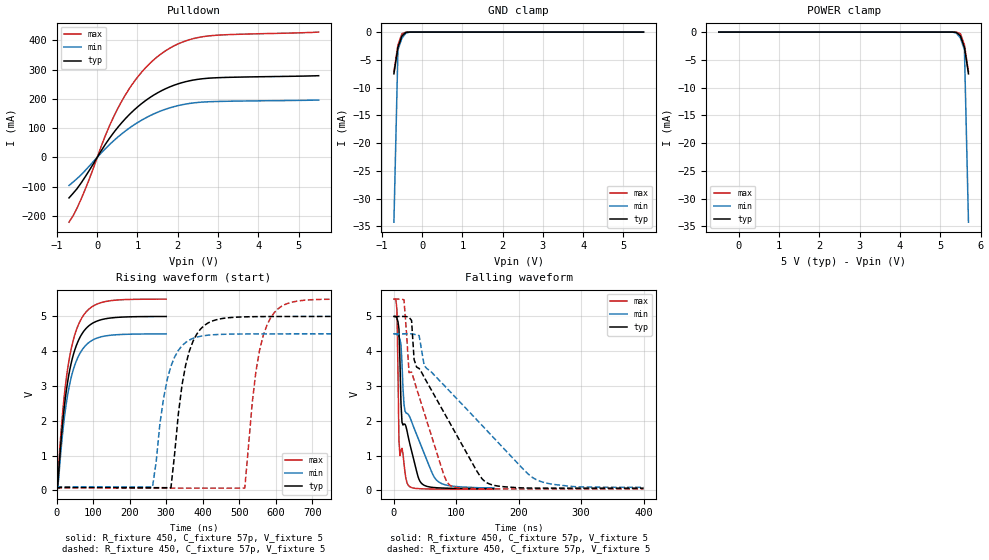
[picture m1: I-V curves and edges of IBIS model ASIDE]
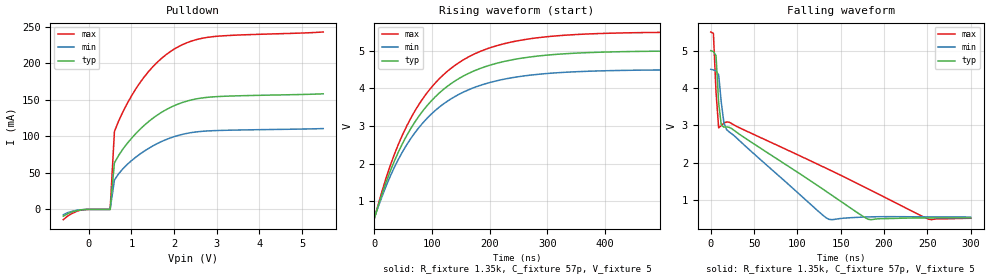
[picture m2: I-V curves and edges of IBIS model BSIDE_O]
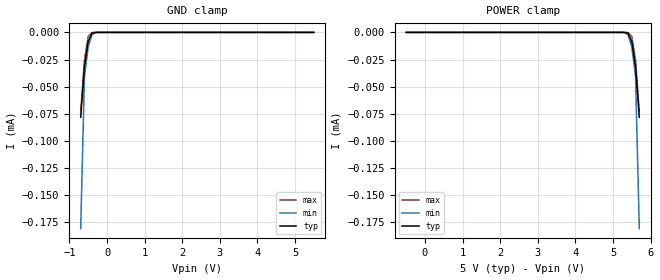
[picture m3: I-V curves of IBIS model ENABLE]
[IBIS Ver]   3.2
[Comment Char]   |_char
| VDD nom: 5v, min: 4.5v, max:5.5v
[File name]   pca9507_a_5.ibs
[File Rev]   1
[Date]   Sep 19, 2008 3:12:36 PM
[Source]
Generated using IBISToolkit at NXP Tempe by Seshadri Venkataramanan
[Notes]
[Disclaimer]
(C) Copyright 2007 NXP Semiconductors
All rights reserved
NXP Semiconductors (NXP) does not warrant that this model and any other
accompanying information (Model) accurately or fully represents the
operating characteristics and specifications of the semiconductor
products to which the Model relates.  Moreover, the Model is furnished
on an "as is" and with "all faults" basis, and without support or
warranty of any kind.  NXP disclaims all warranties, whether expressed
or implied or statutory, including without limitation all implied
warranties of non-infringement, merchantability and fitness for any
purpose, and those arising from a course of dealing or usage of trade.
NXP does not convey any license under its or any third party's patents,
copyrights or other intellectual property or proprietary rights.
You and your company assume any and all risks and liability arising out
of the application or use of the Model.
In no event shall NXP be liable for any direct, indirect, special,
consequential or incidental damages, however caused, whether in
warranty, contract or tort (including negligence), strict liability or
other legal theory, including, without limitation, for lost profits,
business interruption, or corruption or loss of data or information,
arising out of or in connection with the use of or the inability to use
the Model, even if NXP has been advised of the possibility of such
damages.
NXP provides the Model as a courtesy to our customers. You and your
company shall not distribute, convey, sell, or give the Model to anyone
else without receiving prior written permission from NXP.
NXP reserves the right to make changes without notice to the Model to
improve reliability, function, or design.
Please be aware that your receipt and subsequent use of the Model shall
serve as acceptance of these terms and conditions.  If you do not
accept these terms, return or destroy the Model immediately.
[Copyright]
2008
| SO8
[Component]   PCA9507D
Si_location Pin
Timing_location Pin
[Manufacturer]   NXP
[Package]
R_pkg   4.81E-02   4.14E-02   5.47E-02
L_pkg   1.88n   1.54n   2.21n
C_pkg   4.49E-13   4.17E-13   4.81E-13
[Pin] signal_name   model_name   R_pin   L_pin   C_pin
1   VCCA   POWER   5.47E-02  2.21E-09  4.81E-13
2   SCLA   ASIDE   4.14E-02  1.54E-09  4.20E-13
3   SDAA   ASIDE   4.14E-02  1.55E-09  4.20E-13
4   GND   GND   5.47E-02  2.21E-09  4.80E-13
5   EN   ENABLE   5.47E-02  2.21E-09  4.78E-13
6   SDAB   BSIDE_I/O   4.14E-02  1.55E-09  4.17E-13
7   SCLB   BSIDE_I/O   4.14E-02  1.54E-09  4.17E-13
8   VCCB   POWER   5.47E-02  2.21E-09  4.79E-13
| TSSOP8
[Component]   PCA9507AD
Si_location Pin
Timing_location Pin
[Manufacturer]   NXP
[Package]
R_pkg   33.7m   30.1m   37.3m
L_pkg   1.74n   1.67n   1.81n
C_pkg   0.428p   0.422p   0.434p
[Pin] signal_name   model_name   R_pin   L_pin   C_pin
1   VCCA   POWER   37.3m   1.81nH   0.428pF
2   SCLA   ASIDE   30.1m   1.67nH   0.422pF
3   SDAA   ASIDE   30.1m   1.67nH   0.428pF
4   GND   GND   37.3m   1.81nH   0.434pF
5   EN   ENABLE   37.3m   1.81nH   0.428pF
6   SDAB   BSIDE_I/O   30.1m   1.67nH   0.422pF
7   SCLB   BSIDE_I/O   30.1m   1.67nH   0.428pF
8   VCCB   POWER   37.3m   1.81nH   0.434pF
[Model Selector]   BSIDE_I/O
BSIDE_I   Bside as Input
BSIDE_O   Bside as Output
| Models and submodels in the file (4): ASIDE (I/O_open_drain), BSIDE_O (Open_drain), ENABLE (Input), BSIDE_I (Input)
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[Model]   ASIDE
Model_type I/O_open_drain
Vinh=3.5
Vinl=1.5
Vref=5
Vmeas=2.5
Rref=450
Cref=57p
C_comp   5.2p   5p   5.4p
[Temperature Range] 27   85   -40
[Voltage Range]   5   4.5   5.5
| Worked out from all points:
|   slope of the pulldown table from 0 to 0.75 V, typ, clamps not added: 5.37 ohm
|   GND clamp passes 1 mA (typ) near -0.52 V on its own axis
|   falling waveform, R_fixture 450, C_fixture 57p, V_fixture 5: 20-80 % time 20.5ns typ, 37.9ns min, 3.61ns max; typ from 5 V to 0.049 V
|   falling waveform, R_fixture 450, C_fixture 57p, V_fixture 5: 20-80 % time 85.9ns typ, 140ns min, 47.2ns max; typ from 5 V to 0.061 V
|   rising waveform, R_fixture 450, C_fixture 57p, V_fixture 5: 20-80 % time 39.7ns typ, 39.8ns min, 39.6ns max; typ from 0.048 V to 5 V
|   rising waveform, R_fixture 450, C_fixture 57p, V_fixture 5: 20-80 % time 40.5ns typ, 40.9ns min, 40.5ns max; typ from 0.061 V to 5 V
[Pulldown]
-700mV    -138.9mA   -96.33mA   -222.1mA
-600mV    -123.5mA   -84.89mA   -200.6mA
-400mV    -87.94mA   -59.92mA   -143mA
-200mV    -45.56mA   -30.51mA   -75.7mA
200mV     44.01mA    29.24mA    73.36mA
600mV     117mA      79.31mA    190.1mA
800mV     146.6mA    100.3mA    235.7mA
1.1V      183.6mA    126.9mA    291mA
1.6V      228.3mA    159.8mA    355.5mA
2.1V      255.4mA    179.8mA    393.6mA
2.7V      270.2mA    189.8mA    414.5mA
5.5V      279.4mA    196.1mA    428.8mA
[GND Clamp]
-700mV    -7.514mA   -34.24mA   -7.128mA
-600mV    -2.754mA   -3.204mA   -2.306mA
-500mV    -688.4uA   -1.069mA   -295.4uA
-400mV    -56.78uA   -166.7uA   -8.032uA
-200mV    -26.65nA   -203.8nA   -760.1pA
5.5V      375pA      669.7pA    343.7pA
[POWER Clamp]
-500mV    375pA      669.7pA    343.7pA
5.2V      -26.65nA   -203.8nA   -760.1pA
5.4V      -56.78uA   -166.7uA   -8.032uA
5.5V      -688.4uA   -1.069mA   -295.4uA
5.6V      -2.754mA   -3.204mA   -2.306mA
5.7V      -7.514mA   -34.24mA   -7.128mA
[Falling Waveform]
R_fixture=450
C_fixture=57p
V_fixture=5
V_fixture_min=4.5
V_fixture_max=5.5
0s        5V         4.5V       5.5V
4.848ns   4.951V     4.489V     5.198V
8.081ns   4.643V     4.412V     1.43V
9.697ns   3.689V     4.343V     994mV
12.93ns   1.961V     3.654V     1.206V
16.16ns   1.905V     2.473V     768mV
22.63ns   1.566V     2.192V     153.7mV
42.02ns   250.3mV    1.352V     45.07mV
69.49ns   72.05mV    272.6mV    34.02mV
160ns     48.56mV    67.26mV    32.13mV
[Falling Waveform]
R_fixture=450
C_fixture=57p
V_fixture=5
V_fixture_min=4.5
V_fixture_max=5.5
0s        5V         4.5V       5.5V
16.16ns   5V         4.5V       5.477V
24.24ns   4.976V     4.5V       3.385V
28.28ns   4.886V     4.499V     3.401V
36.36ns   3.543V     4.471V     2.919V
48.48ns   3.251V     3.591V     2.235V
88.89ns   1.96V      2.859V     155.3mV
153.5ns   178.3mV    1.631V     39.97mV
234.3ns   62.63mV    258.8mV    39.21mV
400ns     61.43mV    86.93mV    39.15mV
[Rising Waveform]
R_fixture=450
C_fixture=57p
V_fixture=5
V_fixture_min=4.5
V_fixture_max=5.5
0s        48.39mV    65.64mV    32.09mV
3.03ns    88.66mV    71.06mV    214.1mV
9.091ns   990.4mV    766.2mV    1.213V
18.18ns   2.093V     1.787V     2.399V
30.3ns    3.111V     2.736V     3.484V
48.48ns   3.985V     3.554V     4.417V
69.7ns    4.499V     4.033V     4.964V
93.94ns   4.773V     4.289V     5.253V
130.3ns   4.924V     4.431V     5.419V
300ns     4.997V     4.497V     5.496V
[Rising Waveform]
R_fixture=450
C_fixture=57p
V_fixture=5
V_fixture_min=4.5
V_fixture_max=5.5
0s        61.32mV    86.34mV    39.12mV
262.6ns   74.93mV    94.31mV    62.76mV
292.9ns   74.46mV    2.642V     62.1mV
313.1ns   74.36mV    3.569V     61.88mV
343.4ns   3.029V     4.156V     61.72mV
373.7ns   4.292V     4.37V      61.64mV
515.2ns   4.987V     4.495V     61.51mV
545.5ns   4.993V     4.496V     3.404V
596ns     4.997V     4.498V     5.111V
1us       4.999V     4.499V     5.498V
[Ramp]
R_load=450
dV/dt_r   2.970E+0/2.647E-9   2.955E+0/2.392E-9   2.981E+0/3.067E-9
dV/dt_f   2.971E+0/1.933E-8   2.956E+0/4.536E-8   2.982E+0/3.815E-9
|[End   ASIDE
[Model]   BSIDE_O
Model_type Open_drain
Vref=5
Vmeas=2.5
Rref=1.35k
Cref=57p
C_comp   4.8p   4.6p   5p
[Temperature Range] 27   85   -40
[Voltage Range]   5   4.5   5.5
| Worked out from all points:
|   slope of the pulldown table from 0 to 0.75 V, typ, clamps not added: 9.58 ohm
|   falling waveform, R_fixture 1.35k, C_fixture 57p, V_fixture 5: 20-80 % time 114ns typ, 81.9ns min, 158ns max; typ from 5 V to 0.519 V
|   rising waveform, R_fixture 1.35k, C_fixture 57p, V_fixture 5: 20-80 % time 112ns typ, 113ns min, 112ns max; typ from 0.523 V to 5 V
[Pulldown]
-600mV    -9.215mA   -7.302mA   -14.07mA
-400mV    -3.613mA   -2.726mA   -5.734mA
-200mV    -741.7uA   -580uA     -1.156mA
500mV     7.249uA    5.859uA    4.864uA
600mV     63.63mA    40.28mA    106.5mA
900mV     90.25mA    61.55mA    144.9mA
1.2V      109.6mA    75.72mA    173.4mA
1.5V      124.7mA    86.82mA    195.1mA
1.9V      139.1mA    97.52mA    215.5mA
2.3V      148.2mA    104mA      228mA
2.8V      153.5mA    107.4mA    235.6mA
5.5V      158.2mA    110.6mA    242.8mA
[Falling Waveform]
R_fixture=1.35k
C_fixture=57p
V_fixture=5
V_fixture_min=4.5
V_fixture_max=5.5
0s        5V         4.5V       5.5V
3.03ns    4.975V     4.483V     5.462V
6.061ns   4.866V     4.452V     3.889V
9.091ns   3.599V     4.351V     2.932V
12.12ns   3.007V     3.617V     2.99V
18.18ns   2.957V     2.886V     3.089V
133.3ns   1.227V     518.8mV    1.847V
181.8ns   482.4mV    545.7mV    1.294V
251.5ns   519.6mV    546.8mV    485.4mV
300ns     518.5mV    542.9mV    510mV
[Rising Waveform]
R_fixture=1.35k
C_fixture=57p
V_fixture=5
V_fixture_min=4.5
V_fixture_max=5.5
0s        522.8mV    547.9mV    512.6mV
21.21ns   1.52V      1.418V     1.636V
35.35ns   2.076V     1.909V     2.254V
70.71ns   3.106V     2.821V     3.4V
91.92ns   3.543V     3.207V     3.885V
120.2ns   3.973V     3.587V     4.363V
176.8ns   4.487V     4.041V     4.935V
240.4ns   4.762V     4.287V     5.239V
332.3ns   4.921V     4.429V     5.413V
700ns     4.998V     4.498V     5.498V
[Ramp]
R_load=1350
dV/dt_r   2.685E+0/7.049E-9   2.669E+0/7.001E-9   2.692E+0/7.042E-9
dV/dt_f   2.689E+0/1.066E-7   2.674E+0/9.433E-8   2.693E+0/1.147E-7
|[End   BSIDE_O
[Model]   ENABLE
Model_type Input
Vinh=3.5
Vinl=1.5
C_comp   1.7p   1.5p   1.9p
[Temperature Range] 27   85   -40
[Voltage Range]   5   4.5   5.5
[GND Clamp]
-700mV    -78.2uA    -180.8uA   -72.93uA
-600mV    -31.83uA   -40.84uA   -25.27uA
-500mV    -8.452uA   -13.3uA    -3.68uA
-400mV    -758.4nA   -2.213uA   -96.83nA
-300mV    -18.6nA    -106.4nA   -805pA
-200mV    -273.4pA   -2.436nA   -5.553pA
5.5V      11.09pA    12.98pA    11pA
[POWER Clamp]
-500mV    11.09pA    12.98pA    11pA
5.2V      -273.4pA   -2.436nA   -5.553pA
5.3V      -18.6nA    -106.4nA   -805pA
5.4V      -758.4nA   -2.213uA   -96.83nA
5.5V      -8.452uA   -13.3uA    -3.68uA
5.6V      -31.83uA   -40.84uA   -25.27uA
5.7V      -78.2uA    -180.8uA   -72.93uA
